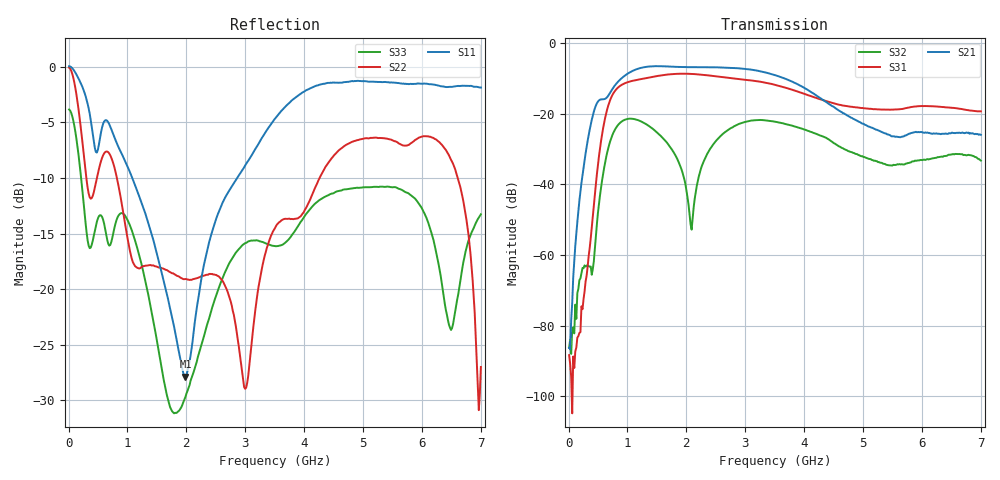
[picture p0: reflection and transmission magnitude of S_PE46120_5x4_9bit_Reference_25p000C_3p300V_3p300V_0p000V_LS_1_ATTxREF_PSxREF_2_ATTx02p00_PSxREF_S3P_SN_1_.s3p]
! Device ID: PE46120_5x4_9bit_Reference
! Device ID: PE46120_5x4_9bit_Reference
! File Path: z:\PE46120_5x4_9bit_Reference\MPAC_Yi\new_12port\25p000C\3p300\LS_1_ATTxREF_PSxREF_2_ATTx02p00_PSxREF\PE46120_5x4_9bit_Reference_25p000C_3p300V_3p300V_0p000V_LS_1_ATTxREF_PSxREF_2_ATTx02p00_PSxREF_S3P_SN_1_.s3p
! Serial: 1
! Lot:
! Temp: 25.000C
! VDD: 3.300
! VSS: 0.000
! Control_Hi: 3.300
! Control_Lo: 0.000
! Logic State: LS_1_ATTxREF_PSxREF_2_ATTx02p00_PSxREF
! Port 1: RFin
! Port 2: RFout1
! Port 3: RFout2
! ThroughPath:1-3
! IDD: -0.0005459313
! ISS: 0
! Comment:
#  Hz  S  RI  R  50
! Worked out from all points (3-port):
!   401 points, 10 MHz to 7 GHz, reference 50 ohm
!   strongest paths, dB at 10 MHz, 1.758 GHz, 3.505 GHz, 5.253 GHz, 7 GHz:
!     S21: -86.3, -6.7, -9.1, -24.7, -26.0
!     S31: -88.4, -8.8, -11.8, -18.8, -19.3
!     S32: -86.2, -30.2, -22.2, -33.7, -33.3
!   lowest |S11| = -27.9 dB at 1.985 GHz (marker M1), VSWR 1.08, Z = 53.4 + j2.4 ohm
!   |S11| at or under -10 dB: 1.082 GHz to 2.862 GHz (1.78 GHz wide, 90.2 % of centre)
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1e7  1.001 -0.1153  -0.000122 7.35e-05  2.02e-06 -8.15e-05
     3.34e-05 3.52e-05  0.987 -0.0964  7.36e-05 -6.66e-06
     3.48e-05 -1.57e-05  2.14e-06 -4.87e-05  0.6399 -0.0623
2.37175e8  -0.4726 -0.6579  -0.0127 -0.00501  1.55e-06 0.000237
           -0.0125 -0.00501  -0.2891 -0.3519  -0.000233 0.00057
           6.41e-05 0.000158  -0.000223 0.000614  -0.1689 -0.2166
4.6435e8  -0.4076 -0.0723  -0.0568 0.1163  0.00954 0.00301
          -0.0571 0.1178  0.1371 0.2681  -0.00135 0.0013
          0.00959 0.00304  -0.00139 0.00126  0.1096 0.1587
9.36175e8  -0.292 0.257  0.3299 -0.0456  -0.0953 0.245
           0.3337 -0.0465  -0.0449 -0.2104  -0.0483 0.064
           -0.0956 0.2479  -0.0486 0.0647  0.0905 -0.1981
1.984675e9  0.0336 0.0224  -0.3663 0.2666  -0.2228 -0.2889
            -0.37 0.2701  -0.09 0.0651  0.00169 0.00948
            -0.2265 -0.2916  0.00174 0.00989  -0.0326 -0.00332
2.823475e9  -0.0925 -0.2899  0.4339 0.072  -0.0652 0.3033
            0.4388 0.0717  0.0652 -0.031  0.0149 0.0651
            -0.065 0.3071  0.0147 0.0657  0.0525 0.1337
3.505e9  -0.4306 -0.3959  -0.092 -0.3358  0.252 0.0342
         -0.0931 -0.34  0.0622 0.1777  0.00748 -0.0757
         0.2552 0.034  0.00698 -0.077  0.1097 -0.1114
4.58845e9  -0.8466 0.0505  -0.0123 0.1092  -0.0491 -0.1235
           -0.0121 0.1106  -0.3987 0.1364  0.0218 0.0269
           -0.0503 -0.1248  0.0222 0.0267  -0.1953 0.1955
6.26605e9  -0.3673 0.7397  0.0391 -0.0332  -0.00611 0.125
           0.0395 -0.0341  0.4517 -0.1084  -0.0243 -0.00278
           -0.00523 0.1264  -0.0242 -0.00253  0.1251 -0.0524
7e9  -0.1086 0.7999  -0.0288 -0.04  0.0963 0.045
     -0.0304 -0.0401  -0.0372 0.0247  0.0199 0.00852
     0.0984 0.0453  0.02 0.00857  0.0998 0.193
